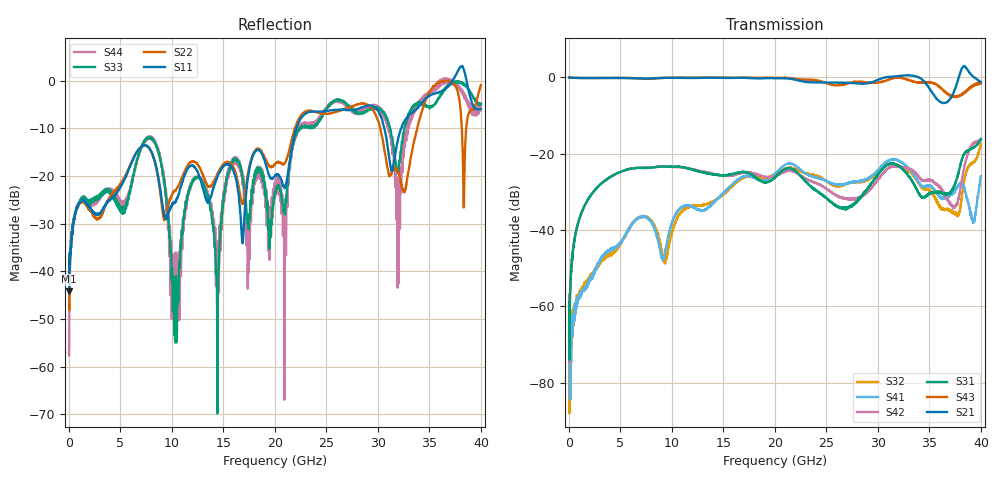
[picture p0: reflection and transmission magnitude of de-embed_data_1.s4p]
!Keysight Technologies,N5225B,MY51451420,A.15.40.08
!Date: Monday, July 18, 2022 07:50:08
!Correction: S11(C  4-Port  )
!S12(C  4-Port  )
!S13(C  4-Port  )
!S14(C  4-Port  )
!S21(C  4-Port  )
!S22(C  4-Port  )
!S23(C  4-Port  )
!S24(C  4-Port  )
!S31(C  4-Port  )
!S32(C  4-Port  )
!S33(C  4-Port  )
!S34(C  4-Port  )
!S41(C  4-Port  )
!S42(C  4-Port  )
!S43(C  4-Port  )
!S44(C  4-Port  )
!S4P File: Measurements: <S11,S12,S13,S14>,
!<S21,S22,S23,S24>,
!<S31,S32,S33,S34>,
!<S41,S42,S43,S44>:
# Hz S  dB  R 50
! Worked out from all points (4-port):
!   4000 points, 10 MHz to 40 GHz, reference 50 ohm
!   strongest paths, dB at 10 MHz, 10.01 GHz, 20.01 GHz, 30.01 GHz, 40 GHz:
!     S21: -0.1, -0.2, -0.3, -0.7, -1.3
!     S43: -0.1, -0.1, -0.1, -1.4, -1.5
!     S31: -62.3, -23.4, -26.2, -25.5, -16.1
!     S42: -57.0, -23.5, -25.9, -26.7, -16.3
!     S41: -67.2, -38.0, -25.2, -24.3, -25.9
!     S32: -67.4, -40.4, -25.4, -24.6, -17.5
!   lowest |S11| = -44.2 dB at 10 MHz (marker M1), VSWR 1.01, Z = 49.5 - j0.339 ohm
!   |S11| at or under -10 dB: start of sweep to 22.08 GHz; 30.63 GHz to 32.26 GHz (1.637 GHz wide, 5.21 % of centre)
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1e7  -44.22 -146.1  -0.08 -0.3  -67.84 117.3  -62.87 111.3
     -0.08 -0.1  -46.99 134.6  -59.91 61.7  -61.23 132.0
     -62.25 -100.2  -67.37 93.2  -40.41 -145.9  -0.08 0.1
     -67.21 -93.3  -56.96 -173.8  -0.06 -0.2  -57.63 71.1
9.03e9  -25.36 -71.5  -0.16 -176.6  -23.37 -81.1  -47.26 48.8
        -0.16 -176.6  -26.48 -102.7  -45.47 25.5  -23.36 -84.1
        -23.38 -81.1  -45.26 26.2  -18.19 -78.0  -0.20 -168.1
        -47.46 46.2  -23.35 -84.2  -0.18 -168.2  -17.50 -73.5
1.036e10  -25.36 -50.3  -0.16 156.2  -23.39 -107.1  -35.94 72.1
          -0.15 156.1  -23.01 179.9  -37.74 78.5  -23.52 -110.3
          -23.39 -107.0  -37.71 78.6  -48.06 0.3  -0.11 165.5
          -35.84 71.7  -23.51 -110.3  -0.11 165.4  -38.90 88.1
1.834e10  -14.51 46.7  -0.31 -9.2  -26.61 84.5  -26.78 -97.4
          -0.30 -9.3  -14.25 108.2  -26.19 -98.6  -25.52 79.2
          -26.66 84.1  -26.18 -98.9  -19.15 75.9  -0.14 6.2
          -26.77 -97.3  -25.51 79.1  -0.14 6.1  -19.09 96.2
3.052e10  -9.27 166.3  -0.17 78.3  -23.74 27.5  -22.89 22.0
          -0.16 78.2  -13.04 -171.1  -23.43 12.7  -25.10 23.6
          -23.76 27.1  -23.42 12.9  -6.51 -173.0  -1.10 101.6
          -22.86 21.7  -25.03 23.2  -1.10 101.4  -7.05 -157.1
3.787e10  2.44 166.8  0.14 -88.5  -24.45 -152.9  -28.16 -154.8
          0.14 -88.8  -3.49 151.1  -35.82 -123.1  -31.43 -150.7
          -24.55 -153.6  -35.63 -121.7  -0.18 -164.6  -4.87 -81.1
          -28.12 -156.5  -31.16 -150.7  -4.86 -81.2  -1.17 -167.0
4e10  -5.93 33.3  -1.28 159.7  -16.13 100.4  -26.12 -33.8
      -1.29 159.5  -0.96 101.2  -17.40 9.4  -16.34 134.5
      -16.15 100.6  -17.46 9.9  -4.91 88.3  -1.56 -125.2
      -25.94 -34.5  -16.29 134.7  -1.54 -125.4  -4.79 156.3
